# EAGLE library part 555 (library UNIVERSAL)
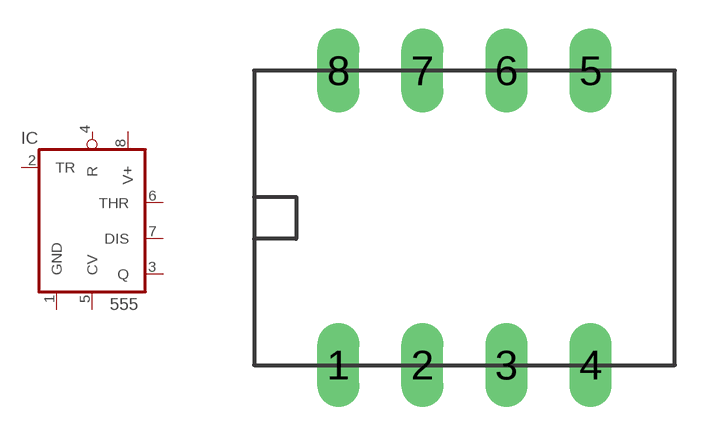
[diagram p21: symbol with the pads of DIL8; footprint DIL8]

Designator prefix IC

## 555  [DIL8]
1  GND  pwr
2  TR  in
3  Q  out
4  R  in
5  CV  in
6  THR  in
7  DIS  in
8  V+  pwr

## Footprint DIL8 (pad centres in mm)
drill 0.61 pad 1.27 long: 1 0,0; 2 2.54,0; 3 5.08,0; 4 7.62,0; 5 7.62,8.89; 6 5.08,8.89; 7 2.54,8.89; 8 0,8.89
